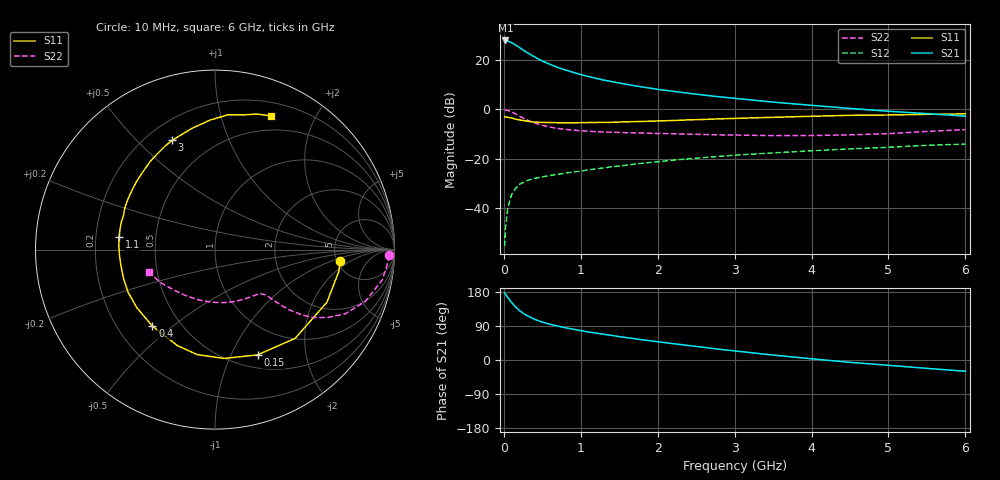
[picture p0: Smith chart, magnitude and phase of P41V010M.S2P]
! SIEMENS Small Signal Semiconductors
! BFP182
! Si NPN RF Bipolar Junction Transistor in SOT143
! VCE = 1 V  IC = 10 mA
! Common Emitter S-Parameters:  March  1996
# GHz  S  MA  R  50
!  f  S11  S21  S12  S22
! GHz  MAG  ANG  MAG  ANG  MAG  ANG  MAG  ANG
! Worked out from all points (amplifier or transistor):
!   36 points, 10 MHz to 6 GHz, reference 50 ohm
!   highest |S21| = 27.9 dB at 20 MHz (marker M1)
!   |S21| within 3 dB of that: start of sweep to 210.3 MHz
!   unconditionally stable (mu >= 1): 936.2 MHz to end of sweep
!   at 250 MHz: K = 0.37, MSG = 26.8 dB, |S12| = -29.7 dB
!   at 1.4 GHz: K = 1.19, MAG = 14.7 dB, |S12| = -23.3 dB
!   at 6 GHz: K = 1.03, MAG = 4.7 dB, |S12| = -14.1 dB
!   S11 on the Smith chart (normalised r, x): 10 MHz: 5.35, -1.31; 150 MHz: 0.65, -1.27; 400 MHz: 0.35, -0.43; 1.1 GHz: 0.30, +0.06; 3 GHz: 0.30, +0.64; 6 GHz: 0.34, +1.45
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0.01  0.7006 -5.1  24.66 177.1  0.0017 87.5  0.9698 -1.9
0.02  0.7004 -10.0  24.7 174.5  0.0037 88.2  0.9666 -4.1
0.05  0.6893 -25.2  24.2 165.2  0.0099 81.6  0.9479 -10.2
0.1  0.6662 -48.0  22.28 151.8  0.0188 68.0  0.8852 -19.1
0.15  0.6326 -68.0  20.09 140.4  0.0248 59.4  0.8093 -26.2
0.2  0.6086 -85.3  17.95 130.9  0.0301 54.0  0.7325 -31.1
0.25  0.5936 -99.5  15.82 123.3  0.0329 49.4  0.665 -34.7
0.3  0.5745 -111.3  14.15 117.3  0.0359 47.0  0.6087 -36.8
0.4  0.551 -129.2  11.45 107.4  0.04 42.9  0.5284 -39.2
0.5  0.5427 -143.5  9.472 100.1  0.043 41.2  0.4731 -40.2
0.6  0.5393 -153.8  8.138 94.3  0.0457 41.1  0.4353 -40.8
0.7  0.5345 -162.3  7.022 89.5  0.0483 41.1  0.41 -41.1
0.8  0.5314 -169.6  6.247 85.1  0.051 41.4  0.3918 -41.5
1  0.536 177.8  5.033 77.5  0.056 42.1  0.3681 -42.6
1.1  0.5394 172.4  4.611 73.9  0.0596 42.1  0.3599 -43.5
1.5  0.5523 155.9  3.397 61.7  0.0713 43.2  0.3399 -48.1
2.2  0.5927 132.1  2.308 43.1  0.0934 41.1  0.3201 -60.2
3  0.6539 111.4  1.668 24.0  0.1177 36.0  0.3007 -79.0
3.5  0.6879 100.7  1.398 13.0  0.1311 32.3  0.294 -92.8
4.5  0.755 84.4  1.041 -6.2  0.158 24.5  0.3035 -122.4
5.5  0.7912 72.7  0.817 -22.1  0.1867 16.9  0.3565 -149.2
6  0.808 67.1  0.726 -29.7  0.1976 12.0  0.3884 -161.4
